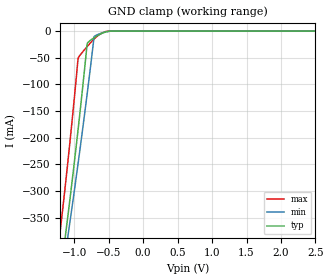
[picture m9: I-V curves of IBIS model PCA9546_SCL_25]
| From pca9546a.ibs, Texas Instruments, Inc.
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[Model]   PCA9546_SCL_25
Model_type  Terminator
| variable   typ   min   max
C_comp   7.10pF   5.50pF   7.78pF
| C_tri-state   7.10pF   5.50pF   7.78pF
[Temperature Range]   40   100   -40
| Ambient temperature   25   85   -40
[Voltage range]   2.5   2.3   2.7
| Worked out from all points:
|   GND clamp passes 1 mA (typ) near -0.52 V on its own axis
[GND Clamp]
| PCA9546_SCL_25
|   Voltage   I(typ)   I(min)   I(max)
-5.5V     -3.656A    -3.511A    -3.814A
-1.215V   -469.9mA   -491.5mA   -387.7mA
-1.17V    -425.8mA   -453mA     -337mA
-1.125V   -380.5mA   -413.8mA   -284.5mA
-1.1V     -354.8mA   -391.7mA   -254.5mA
-1.075V   -328.7mA   -369.3mA   -223.8mA
-945mV    -185.6mA   -249mA     -52.16mA
-810mV    -22.62mA   -115.3mA   -28.77mA
-710mV    -12.38mA   -10.09mA   -14.56mA
-590mV    -3.755mA   -3.176mA   -3.078mA
-495mV    -271.4uA   -426.3uA   -46.53uA
2.5V      243.2pA    746.1pA    146.2pA
